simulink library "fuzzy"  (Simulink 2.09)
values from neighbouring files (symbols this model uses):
  a = -1    [HdataM.m]
  alpha = 4    [VdataM.m]
  b = 1    [HdataM.m]
  ce_n = [-1 -0.5 0 0.5 1]    [HdataF.m]    (also in Mdata.m = e_n; Mdata25.m = e_n; VdataF.m = e_n; VdataF25.m = e_n)
  ceNorm = 0.033    [HdataF.m]    (also in Mdata.m = 1; Mdata25.m = 1; VdataF.m = 0.2; VdataF25.m = 0.2)
  e_n = [-1 -0.5 0 0.5 1]    [HdataF.m]    (also in Mdata.m = [-1 -0.25 0 0.25 1]; Mdata25.m = [-1 -0.5 -0.25 0 0.25 0.5 1]; VdataF.m = [-1 -0.25 0 0.25 1]; VdataF25.m = [-1 -0.5 -0.25 0 0.25 0.5 1])
  eNorm = 0.033    [HdataF.m]    (also in Mdata.m = 1; Mdata25.m = 1; VdataF.m = 0.1; VdataF25.m = 0.1)
  Fe0 = Fi+gamma*sqrt(theta0)    [VdataM.m]
  Fg = 0    [VdataM.m]
  Fi = 1000    [VdataM.m]
  gamma = 12500    [VdataM.m]
  gamma1 = 0    [VdataM.m]
  gamma3 = 0    [VdataM.m]
  LN = [1 1 0 0 0 0 0]    [Mdata25.m]    (also in VdataF25.m)
  LP = [0 0 0 0 0 1 1]    [Mdata25.m]    (also in VdataF25.m)
  m = 1000    [VdataM.m]
  N = [1 1 0 0 0]    [HdataF.m]    (also in Mdata.m; VdataF.m)
  P = [0 0 0 1 1]    [HdataF.m]    (also in Mdata.m; VdataF.m)
  Qt = 10    [HdataM.m]
  SN = [0 0 1 0 0 0 0]    [Mdata25.m]    (also in VdataF25.m)
  SP = [0 0 0 0 1 0 0]    [Mdata25.m]    (also in VdataF25.m)
  T = 2.5    [HdataF.m]    (also in Mdata.m = 0.5; Mdata25.m = 0.5; VdataC.m = 0.25; VdataF.m = 0.25)
  T0 = 50    [HdataM.m]
  Tc = 0    [HdataM.m]
  te_n = 0.1    [VdataM.m]
  te_p = 1    [VdataM.m]
  Th = 100    [HdataM.m]
  theta0 = ((1/gamma)*(alpha*v0^2-Fi))^2    (= 0.186624)    [VdataM.m]
  thetamax = pi/3    (= 1.0471975512)    [VdataM.m]
  u0 = 0    [HdataF.m]    (also in Mdata.m; Mdata25.m; VdataF.m = theta0; VdataF25.m = theta0)
  uDenorm = 0.05    [HdataF.m]    (also in Mdata.m = 1; Mdata25.m = 1; VdataF.m = 0.1; VdataF25.m = 0.1)
  uLN = -1    [Mdata25.m]    (also in VdataF25.m)
  uLP = 1    [Mdata25.m]    (also in VdataF25.m)
  uN = -1    [Mdata.m]    (also in VdataF.m)
  uP = 1    [Mdata.m]    (also in VdataF.m)
  uSN = -0.5    [Mdata25.m]    (also in VdataF25.m)
  uSP = 0.5    [Mdata25.m]    (also in VdataF25.m)
  uZ = 0    [Mdata.m]    (also in Mdata25.m; VdataF.m; VdataF25.m)
  v0 = 40    [VdataM.m]
  Z = [0 0 1 0 0]    [HdataF.m]    (also in Mdata.m; Mdata25.m = [0 0 0 1 0 0 0]; VdataF.m; VdataF25.m = [0 0 0 1 0 0 0])
undefined symbols (not defined in the file or in its folder): i1, i2, nb, nm, pb, pm, x, ze, zi
libraries: fuzzy x6
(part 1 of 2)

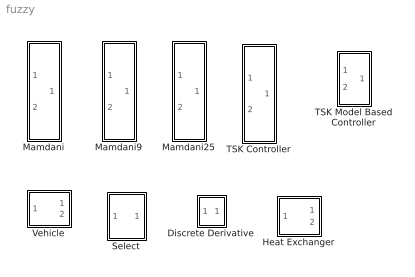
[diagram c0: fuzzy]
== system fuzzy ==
  Discrete Derivative : Subsystem
  Heat Exchanger : Subsystem
  Mamdani : Subsystem
  Mamdani25 : Subsystem
  Mamdani9 : Subsystem
  Select : Subsystem
  TSK Controller : Subsystem
  TSK Model Based Controller : Subsystem
  Vehicle : Subsystem

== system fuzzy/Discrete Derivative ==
  e : Inport  Port=1  PortWidth=-1  SampleTime=-1
  Sum1 : Sum  Inputs=+-
  Unit Delay : UnitDelay  X0=0  SampleTime=T
  ce : Outport  Port=1  InitialOutput=0
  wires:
  e/1 -> Unit Delay/1, Sum1/1
  Sum1/1 -> ce/1
  Unit Delay/1 -> Sum1/2

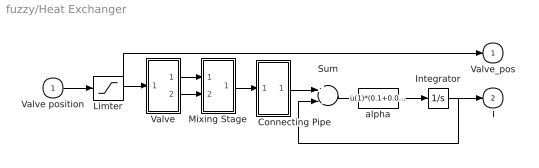
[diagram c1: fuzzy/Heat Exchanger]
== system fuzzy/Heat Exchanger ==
  Valve position : Inport  Port=1  PortWidth=-1  SampleTime=-1
  Connecting Pipe : Subsystem
  Integrator : Integrator  ExternalReset=none  InitialConditionSource=internal  InitialCondition=T0  LimitOutput=off  UpperSaturationLimit=inf  LowerSaturationLimit=-inf  ShowSaturationPort=off  ShowStatePort=off  AbsoluteTolerance=auto
  Limter : Saturate  UpperLimit=1  LowerLimit=-1
  Mixing Stage : Subsystem
  Sum : Sum  Inputs=+-
  Valve : Subsystem
  alpha : Fcn  Expr=u(1)*(0.1+0.01*abs(u(1)))
  Valve_pos : Outport  Port=1  InitialOutput=0
  T : Outport  Port=2  InitialOutput=0
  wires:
  Limter/1 -> Valve_pos/1, Valve/1(Valve_position)
  alpha/1 -> Integrator/1
  Integrator/1 -> T/1, Sum/2
  Valve position/1 -> Limter/1
  Valve/2(Qc) -> Mixing Stage/2(Qc)
  Valve/1(Qh) -> Mixing Stage/1(Qh)
  Mixing Stage/1(Tm) -> Connecting Pipe/1(Tm)
  Sum/1 -> alpha/1
  Connecting Pipe/1(Tf) -> Sum/1

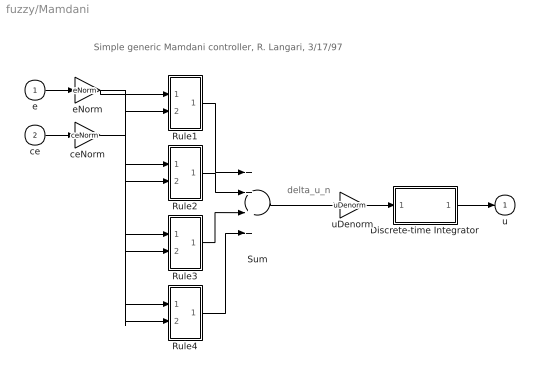
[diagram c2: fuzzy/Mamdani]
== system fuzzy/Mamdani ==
  note: Simple generic Mamdani controller, R. Langari, 3/17/97
  note: delta_u_n
  e : Inport  Port=1  PortWidth=-1  SampleTime=-1
  ce : Inport  Port=2  PortWidth=-1  SampleTime=-1
  Discrete-time Integrator : Subsystem
  Rule1 : Subsystem
  Rule2 : Subsystem
  Rule3 : Subsystem
  Rule4 : Subsystem
  Sum : Sum  Inputs=++++
  ceNorm : Gain  Gain=ceNorm
  eNorm : Gain  Gain=eNorm
  uDenorm : Gain  Gain=uDenorm
  u : Outport  Port=1  InitialOutput=0
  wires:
  ce/1 -> ceNorm/1
  e/1 -> eNorm/1
  eNorm/1 -> Rule2/1(e_n), Rule3/1(e_n), Rule4/1(e_n), Rule1/1(e_n)
  ceNorm/1 -> Rule1/2(ce_n), Rule2/2(ce_n), Rule3/2(ce_n), Rule4/2(ce_n)
  Rule1/1(delta_u_n) -> Sum/1
  Rule2/1(delta_u_n) -> Sum/2
  Rule3/1(delta_u_n) -> Sum/3
  Rule4/1(delta_u_n) -> Sum/4
  Sum/1 -> uDenorm/1
  uDenorm/1 -> Discrete-time Integrator/1(delta_u)
  Discrete-time Integrator/1(u) -> u/1

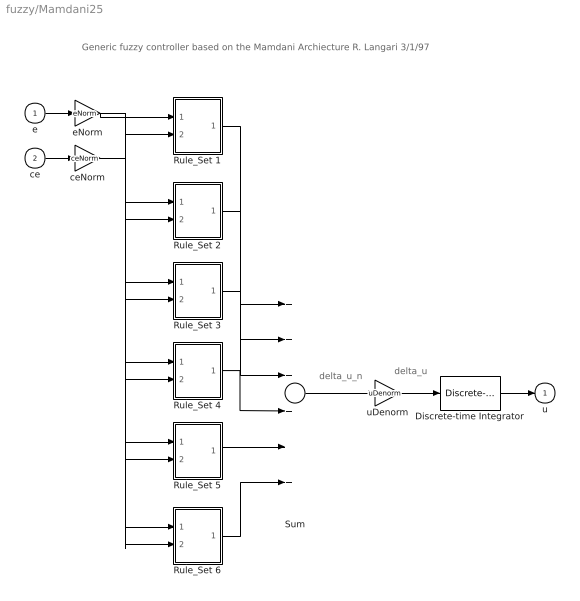
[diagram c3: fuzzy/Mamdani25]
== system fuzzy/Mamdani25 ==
  note: Generic fuzzy controller based on the Mamdani Archiecture R. Langari 3/1/97
  note: delta_u_n
  note: delta_u
  e : Inport  Port=1  PortWidth=-1  SampleTime=-1
  ce : Inport  Port=2  PortWidth=-1  SampleTime=-1
  Discrete-time Integrator : fuzzy/Mamdani/Discrete-time Integrator
  Rule_Set 1 : Subsystem
  Rule_Set 2 : Subsystem
  Rule_Set 3 : Subsystem
  Rule_Set 4 : Subsystem
  Rule_Set 5 : Subsystem
  Rule_Set 6 : Subsystem
  Sum : Sum  Inputs=++++++
  ceNorm : Gain  Gain=ceNorm
  eNorm : Gain  Gain=eNorm
  uDenorm : Gain  Gain=uDenorm
  u : Outport  Port=1  InitialOutput=0
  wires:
  Rule_Set 6/1(delta_u_n) -> Sum/6
  Rule_Set 5/1(delta_u_n) -> Sum/5
  Rule_Set 4/1(delta_u_n) -> Sum/4
  Rule_Set 3/1(delta_u_n) -> Sum/3
  Rule_Set 2/1(delta_u_n) -> Sum/2
  Rule_Set 1/1(delta_u_n) -> Sum/1
  ceNorm/1 -> Rule_Set 5/2(ce_n), Rule_Set 6/2(ce_n), Rule_Set 4/2(ce_n), Rule_Set 3/2(ce_n), Rule_Set 2/2(ce_n), Rule_Set 1/2(ce_n)
  eNorm/1 -> Rule_Set 6/1(e_n), Rule_Set 5/1(e_n), Rule_Set 4/1(e_n), Rule_Set 3/1(e_n), Rule_Set 2/1(e_n), Rule_Set 1/1(e_n)
  uDenorm/1 -> Discrete-time Integrator/1
  Sum/1 -> uDenorm/1
  ce/1 -> ceNorm/1
  e/1 -> eNorm/1
  Discrete-time Integrator/1 -> u/1

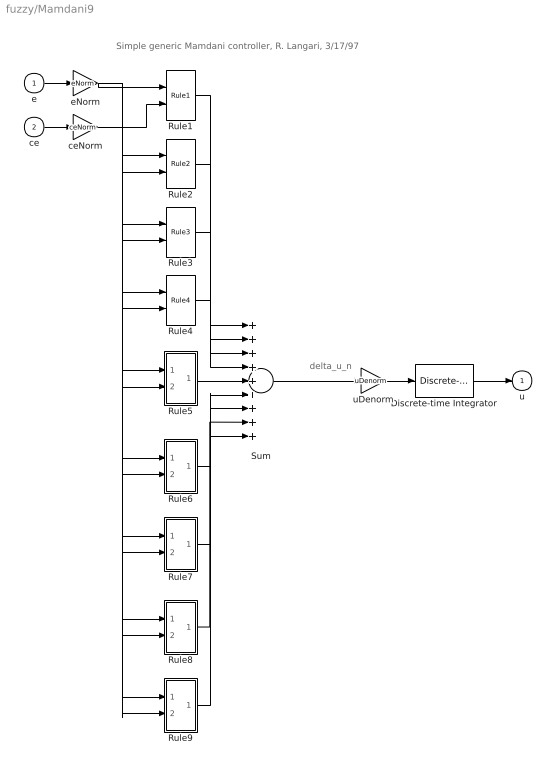
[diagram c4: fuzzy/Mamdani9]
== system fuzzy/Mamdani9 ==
  note: Simple generic Mamdani controller, R. Langari, 3/17/97
  note: delta_u_n
  e : Inport  Port=1  PortWidth=-1  SampleTime=-1
  ce : Inport  Port=2  PortWidth=-1  SampleTime=-1
  Discrete-time Integrator : fuzzy/Mamdani/Discrete-time Integrator
  Rule1 : fuzzy/Mamdani/Rule1
  Rule2 : fuzzy/Mamdani/Rule2
  Rule3 : fuzzy/Mamdani/Rule3
  Rule4 : fuzzy/Mamdani/Rule4
  Rule5 : Subsystem
  Rule6 : Subsystem
  Rule7 : Subsystem
  Rule8 : Subsystem
  Rule9 : Subsystem
  Sum : Sum  Inputs=+++++++++
  ceNorm : Gain  Gain=ceNorm
  eNorm : Gain  Gain=eNorm
  uDenorm : Gain  Gain=uDenorm
  u : Outport  Port=1  InitialOutput=0
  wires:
  Rule4/1 -> Sum/4
  Rule3/1 -> Sum/3
  Rule2/1 -> Sum/2
  Rule1/1 -> Sum/1
  ceNorm/1 -> Rule3/2, Rule2/2, Rule1/2, Rule4/2, Rule5/2(ce_n), Rule6/2(ce_n), Rule7/2(ce_n), Rule8/2(ce_n), Rule9/2(ce_n)
  eNorm/1 -> Rule3/1, Rule2/1, Rule4/1, Rule5/1(e_n), Rule6/1(e_n), Rule7/1(e_n), Rule8/1(e_n), Rule9/1(e_n), Rule1/1
  e/1 -> eNorm/1
  ce/1 -> ceNorm/1
  Rule5/1(delta_u_n) -> Sum/5
  Rule6/1(delta_u_n) -> Sum/6
  Rule7/1(delta_u_n) -> Sum/7
  Rule8/1(delta_u_n) -> Sum/8
  Rule9/1(delta_u_n) -> Sum/9
  uDenorm/1 -> Discrete-time Integrator/1
  Discrete-time Integrator/1 -> u/1
  Sum/1 -> uDenorm/1

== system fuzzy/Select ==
  theta_in : Inport  Port=1  PortWidth=-1  SampleTime=-1
  Manual mode throttle position : Constant  Value=theta0
  On/Off : Constant  Value=1
  Switch : Switch  Threshold=0.5
  theta_out : Outport  Port=1  InitialOutput=0
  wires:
  Switch/1 -> theta_out/1
  theta_in/1 -> Switch/1
  Manual mode throttle position/1 -> Switch/3
  On/Off/1 -> Switch/2

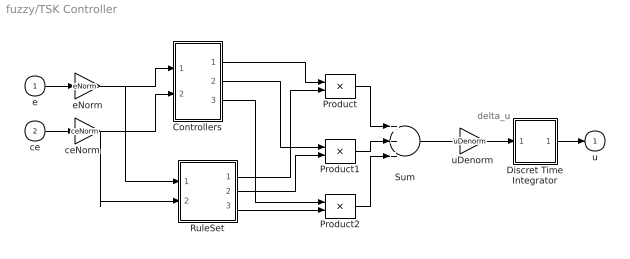
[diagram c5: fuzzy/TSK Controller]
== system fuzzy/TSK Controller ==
  note: delta_u
  e : Inport  Port=1  PortWidth=-1  SampleTime=-1
  ce : Inport  Port=2  PortWidth=-1  SampleTime=-1
  Controllers : Subsystem
  Discret Time Integrator : Subsystem  mask(Discrete-Time Integrator){}
      mask help: Discrete-Time Integrator:
      mask init:
      | X0=@1;Ts=@2;
  Product : Product  Inputs=2
  Product1 : Product  Inputs=2
  Product2 : Product  Inputs=2
  RuleSet : Subsystem
  Sum : Sum  Inputs=+++
  ceNorm : Gain  Gain=ceNorm
  eNorm : Gain  Gain=eNorm
  uDenorm : Gain  Gain=uDenorm
  u : Outport  Port=1  InitialOutput=0
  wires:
  Sum/1 -> uDenorm/1
  Discret Time Integrator/1(out_1) -> u/1
  uDenorm/1 -> Discret Time Integrator/1(in_1)
  ceNorm/1 -> Controllers/2(ce_n), RuleSet/2(ce)
  eNorm/1 -> Controllers/1(e_n), RuleSet/1(e)
  e/1 -> eNorm/1
  ce/1 -> ceNorm/1
  Product1/1 -> Sum/2
  Product/1 -> Sum/1
  RuleSet/2(w2) -> Product1/2
  Controllers/2(delta_u_n2) -> Product1/1
  RuleSet/1(w1) -> Product/2
  Controllers/1(delta_u_n1) -> Product/1
  Controllers/3(delta_u_n3) -> Product2/1
  RuleSet/3(w3) -> Product2/2
  Product2/1 -> Sum/3

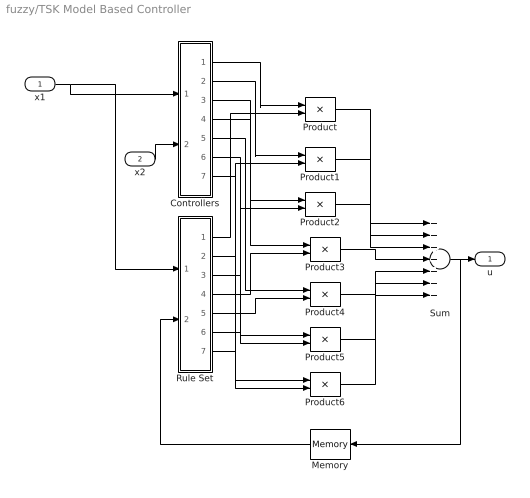
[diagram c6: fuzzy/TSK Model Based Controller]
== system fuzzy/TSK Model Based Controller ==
  x1 : Inport  Port=1  PortWidth=-1  SampleTime=-1
  x2 : Inport  Port=2  PortWidth=-1  SampleTime=-1
  Controllers : Subsystem
  Memory : Memory  Orientation=left  X0=0  InheritSampleTime=off
  Product{,1..6} (7 alike) : Product  Inputs=2
  Rule Set : Subsystem
  Sum : Sum  Inputs=+++++++
  u : Outport  Port=1  InitialOutput=0
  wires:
  Sum/1 -> Memory/1, u/1
  Controllers/1(out_1) -> Product/1
  Rule Set/1(out_1) -> Product/2
  Controllers/2(out_2) -> Product1/1
  Controllers/3(out_3) -> Product2/1
  Controllers/4(out_4) -> Product3/1
  Controllers/5(out_5) -> Product4/1
  Controllers/6(out_6) -> Product5/1
  Controllers/7(out_7) -> Product6/1
  Rule Set/2(out_2) -> Product1/2
  Rule Set/3(out_3) -> Product2/2
  Rule Set/4(out_4) -> Product3/2
  Rule Set/5(out_5) -> Product4/2
  Rule Set/6(out_6) -> Product5/2
  Rule Set/7(out_7) -> Product6/2
  Product/1 -> Sum/1
  Product1/1 -> Sum/2
  Product2/1 -> Sum/3
  Product3/1 -> Sum/4
  Product4/1 -> Sum/5
  Product5/1 -> Sum/6
  Product6/1 -> Sum/7
  x1/1 -> Controllers/1(x1), Rule Set/1(x1)
  Memory/1 -> Rule Set/2(x2)
  x2/1 -> Controllers/2(x2)

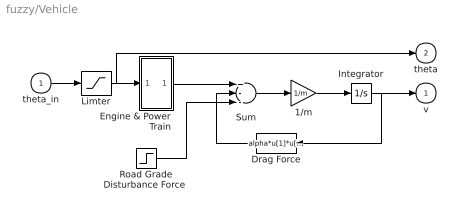
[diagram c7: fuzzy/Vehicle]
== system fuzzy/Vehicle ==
  theta_in : Inport  Port=1  PortWidth=-1  SampleTime=-1
  1/m : Gain  Gain=1/m
  Drag Force : Fcn  Orientation=left  Expr=alpha*u[1]*u[1]
  Engine & Power Train : Subsystem
  Integrator : Integrator  ExternalReset=none  InitialConditionSource=internal  InitialCondition=v0  LimitOutput=off  UpperSaturationLimit=inf  LowerSaturationLimit=-inf  ShowSaturationPort=off  ShowStatePort=off  AbsoluteTolerance=auto
  Limter : Saturate  UpperLimit=thetamax  LowerLimit=0
  "Road Grade Disturbance Force " : Step  Time=0  Before=0  After=Fg
  Sum : Sum  Inputs=+--
  v : Outport  Port=1  InitialOutput=0
  theta : Outport  Port=2  InitialOutput=0
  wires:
  Limter/1 -> theta/1, Engine & Power Train/1(theta)
  "Road Grade Disturbance Force "/1 -> Sum/3
  theta_in/1 -> Limter/1
  Sum/1 -> 1/m/1
  1/m/1 -> Integrator/1
  Integrator/1 -> Drag Force/1, v/1
  Engine & Power Train/1(Engine Force_) -> Sum/1
  Drag Force/1 -> Sum/2

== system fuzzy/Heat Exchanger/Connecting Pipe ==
  Tm : Inport  Port=1  PortWidth=-1  SampleTime=-1
  Integrator : Integrator  ExternalReset=none  InitialConditionSource=internal  InitialCondition=T0  LimitOutput=off  UpperSaturationLimit=inf  LowerSaturationLimit=-inf  ShowSaturationPort=off  ShowStatePort=off  AbsoluteTolerance=auto
  Sum : Sum  Inputs=++
  a : Gain  Orientation=left  Gain=a
  b : Gain  Gain=b
  Tf : Outport  Port=1  InitialOutput=0
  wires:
  a/1 -> Sum/2
  Integrator/1 -> a/1, Tf/1
  b/1 -> Sum/1
  Sum/1 -> Integrator/1
  Tm/1 -> b/1

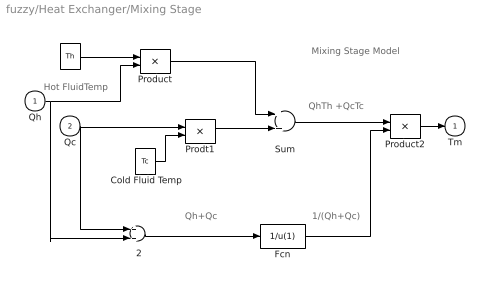
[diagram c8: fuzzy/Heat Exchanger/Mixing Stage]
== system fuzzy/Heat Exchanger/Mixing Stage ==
  note: Mixing Stage Model
  note: 1/(Qh+Qc)
  note: Qh+Qc
  note: QhTh +QcTc
  note: Hot FluidTemp
  Qh : Inport  Port=1  PortWidth=-1  SampleTime=-1
  Qc : Inport  Port=2  PortWidth=-1  SampleTime=-1
  " " : Constant  Value=Th
  " 2" : Sum  Inputs=++
  " Cold Fluid Temp" : Constant  Value=Tc
  Fcn : Fcn  Expr=1/u(1)
  Prodt1 : Product  Inputs=2
  Product : Product  Inputs=2
  Product2 : Product  Inputs=2
  Sum : Sum  Inputs=++
  Tm : Outport  Port=1  InitialOutput=0
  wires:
  Fcn/1 -> Product2/2
  Sum/1 -> Product2/1
  Qh/1 -> " 2"/2, Product/2
  Qc/1 -> " 2"/1, Prodt1/1
  " Cold Fluid Temp"/1 -> Prodt1/2
  " 2"/1 -> Fcn/1
  Prodt1/1 -> Sum/2
  Product/1 -> Sum/1
  " "/1 -> Product/1
  Product2/1 -> Tm/1

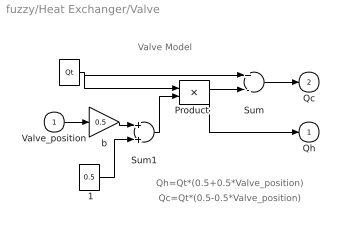
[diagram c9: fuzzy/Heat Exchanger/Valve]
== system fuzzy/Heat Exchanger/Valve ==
  note: Qc=Qt*(0.5-0.5*Valve_position)
  note: Qh=Qt*(0.5+0.5*Valve_position)
  note: Valve Model
  Valve_position : Inport  Port=1  PortWidth=-1  SampleTime=-1
  " " : Constant  Value=Qt
  " 1" : Constant  Value=0.5
  Product : Product  Inputs=2
  Sum : Sum  Inputs=+-
  Sum1 : Sum  Inputs=++
  b : Gain  Gain=0.5
  Qh : Outport  Port=1  InitialOutput=0
  Qc : Outport  Port=2  InitialOutput=0
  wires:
  Sum1/1 -> Product/2
  " 1"/1 -> Sum1/2
  b/1 -> Sum1/1
  Valve_position/1 -> b/1
  Product/1 -> Sum/2, Qh/1
  Sum/1 -> Qc/1
  " "/1 -> Sum/1, Product/1

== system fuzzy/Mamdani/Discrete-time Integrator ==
  delta_u : Inport  Port=1  PortWidth=-1  SampleTime=-1
  Sum : Sum  Inputs=++
  Unit Delay : UnitDelay  Orientation=left  X0=u0  SampleTime=T
  u : Outport  Port=1  InitialOutput=0
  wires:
  Unit Delay/1 -> Sum/2
  Sum/1 -> u/1, Unit Delay/1
  delta_u/1 -> Sum/1

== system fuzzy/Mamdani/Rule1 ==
  note: if e_n is P and ce_n is P then delta_u_n is P
  e_n : Inport  Port=1  PortWidth=-1  SampleTime=-1
  ce_n : Inport  Port=2  PortWidth=-1  SampleTime=-1
  P(ce_n) : Lookup  InputValues=ce_n  OutputValues=P
  P(delta_u_n) : Constant  Value=uP
  P(e_n) : Lookup  InputValues=e_n  OutputValues=P
  Product : Product  Inputs=2
  Product1 : Product  Inputs=2
  delta_u_n : Outport  Port=1  InitialOutput=0
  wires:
  Product/1 -> Product1/1
  ce_n/1 -> P(ce_n)/1
  P(ce_n)/1 -> Product/2
  P(delta_u_n)/1 -> Product1/2
  e_n/1 -> P(e_n)/1
  P(e_n)/1 -> Product/1
  Product1/1 -> delta_u_n/1

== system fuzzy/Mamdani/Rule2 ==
  note: if e_n is P and ce_n is N then delta_u_n is Z
  e_n : Inport  Port=1  PortWidth=-1  SampleTime=-1
  ce_n : Inport  Port=2  PortWidth=-1  SampleTime=-1
  N(ce_n) : Lookup  InputValues=ce_n  OutputValues=N
  P(e_n) : Lookup  InputValues=e_n  OutputValues=P
  Prduct : Product  Inputs=2
  Product1 : Product  Inputs=2
  Z(delta_u_n) : Constant  Value=uZ
  delta_u_n : Outport  Port=1  InitialOutput=0
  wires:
  Product1/1 -> delta_u_n/1
  Z(delta_u_n)/1 -> Product1/2
  Prduct/1 -> Product1/1
  P(e_n)/1 -> Prduct/1
  N(ce_n)/1 -> Prduct/2
  e_n/1 -> P(e_n)/1
  ce_n/1 -> N(ce_n)/1

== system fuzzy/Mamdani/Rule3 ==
  note: if e_n is N and ce_n is P then delta_u_n is Z
  e_n : Inport  Port=1  PortWidth=-1  SampleTime=-1
  ce_n : Inport  Port=2  PortWidth=-1  SampleTime=-1
  N(e_n) : Lookup  InputValues=e_n  OutputValues=N
  P(ce_n) : Lookup  InputValues=ce_n  OutputValues=P
  Product : Product  Inputs=2
  Product1 : Product  Inputs=2
  Z(delta_u_n) : Constant  Value=uZ
  delta_u_n : Outport  Port=1  InitialOutput=0
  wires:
  ce_n/1 -> P(ce_n)/1
  e_n/1 -> N(e_n)/1
  P(ce_n)/1 -> Product/2
  N(e_n)/1 -> Product/1
  Product/1 -> Product1/1
  Z(delta_u_n)/1 -> Product1/2
  Product1/1 -> delta_u_n/1

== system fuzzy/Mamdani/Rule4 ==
  note: if e_n is N and ce_n is N then delta_u_n is N
  e_n : Inport  Port=1  PortWidth=-1  SampleTime=-1
  ce_n : Inport  Port=2  PortWidth=-1  SampleTime=-1
  N(ce_n) : Lookup  InputValues=ce_n  OutputValues=N
  N(delta_u_n) : Constant  Value=uN
  N(e_n) : Lookup  InputValues=e_n  OutputValues=N
  Product : Product  Inputs=2
  Product1 : Product  Inputs=2
  delta_u_n : Outport  Port=1  InitialOutput=0
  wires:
  Product1/1 -> delta_u_n/1
  N(delta_u_n)/1 -> Product1/2
  Product/1 -> Product1/1
  N(e_n)/1 -> Product/1
  N(ce_n)/1 -> Product/2
  e_n/1 -> N(e_n)/1
  ce_n/1 -> N(ce_n)/1

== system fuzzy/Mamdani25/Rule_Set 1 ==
  e_n : Inport  Port=1  PortWidth=-1  SampleTime=-1
  ce_n : Inport  Port=2  PortWidth=-1  SampleTime=-1
  Rule1 : Subsystem
  Rule2 : Subsystem
  Rule3 : Subsystem
  Rule4 : Subsystem
  Sum : Sum  Inputs=++++
  delta_u_n : Outport  Port=1  InitialOutput=0
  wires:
  Sum/1 -> delta_u_n/1
  Rule4/1(delta_u_n) -> Sum/4
  Rule3/1(delta_u_n) -> Sum/3
  Rule2/1(delta_u_n) -> Sum/2
  Rule1/1(delta_u_n) -> Sum/1
  e_n/1 -> Rule4/1(e_n), Rule3/1(e_n), Rule2/1(e_n), Rule1/1(e_n)
  ce_n/1 -> Rule4/2(ce_n), Rule3/2(ce_n), Rule2/2(ce_n), Rule1/2(ce_n)

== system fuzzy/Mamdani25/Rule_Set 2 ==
  e_n : Inport  Port=1  PortWidth=-1  SampleTime=-1
  ce_n : Inport  Port=2  PortWidth=-1  SampleTime=-1
  Rule1 : Subsystem
  Rule2 : Subsystem
  Rule3 : Subsystem
  Rule4 : Subsystem
  Sum : Sum  Inputs=++++
  delta_u_n : Outport  Port=1  InitialOutput=0
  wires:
  Rule1/1(delta_u_n) -> Sum/1
  Rule2/1(delta_u_n) -> Sum/2
  Rule3/1(delta_u_n) -> Sum/3
  Rule4/1(delta_u_n) -> Sum/4
  Sum/1 -> delta_u_n/1
  e_n/1 -> Rule1/1(e_n), Rule2/1(e_n), Rule3/1(e_n), Rule4/1(e_n)
  ce_n/1 -> Rule1/2(ce_n), Rule2/2(ce_n), Rule3/2(ce_n), Rule4/2(ce_n)

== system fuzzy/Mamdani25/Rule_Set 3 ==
  e_n : Inport  Port=1  PortWidth=-1  SampleTime=-1
  ce_n : Inport  Port=2  PortWidth=-1  SampleTime=-1
  Rule1 : Subsystem
  Rule2 : Subsystem
  Rule3 : Subsystem
  Rule4 : Subsystem
  Sum : Sum  Inputs=++++
  delta_u_n : Outport  Port=1  InitialOutput=0
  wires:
  Sum/1 -> delta_u_n/1
  Rule4/1(delta_u_n) -> Sum/4
  Rule3/1(delta_u_n) -> Sum/3
  Rule2/1(delta_u_n) -> Sum/2
  Rule1/1(delta_u_n) -> Sum/1
  e_n/1 -> Rule4/1(e_n), Rule3/1(e_n), Rule2/1(e_n), Rule1/1(e_n)
  ce_n/1 -> Rule4/2(ce_n), Rule3/2(ce_n), Rule2/2(ce_n), Rule1/2(ce_n)

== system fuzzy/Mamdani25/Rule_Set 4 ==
  e_n : Inport  Port=1  PortWidth=-1  SampleTime=-1
  ce_n : Inport  Port=2  PortWidth=-1  SampleTime=-1
  Rule1 : Subsystem
  Rule2 : Subsystem
  Rule3 : Subsystem
  Rule4 : Subsystem
  Sum : Sum  Inputs=++++
  delta_u_n : Outport  Port=1  InitialOutput=0
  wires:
  Rule1/1(delta_u_n) -> Sum/1
  Rule2/1(delta_u_n) -> Sum/2
  Rule3/1(delta_u_n) -> Sum/3
  Rule4/1(delta_u_n) -> Sum/4
  Sum/1 -> delta_u_n/1
  e_n/1 -> Rule1/1(e_n), Rule2/1(e_n), Rule3/1(e_n), Rule4/1(e_n)
  ce_n/1 -> Rule1/2(ce_n), Rule2/2(ce_n), Rule3/2(ce_n), Rule4/2(ce_n)

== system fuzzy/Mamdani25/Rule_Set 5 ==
  e_n : Inport  Port=1  PortWidth=-1  SampleTime=-1
  ce_n : Inport  Port=2  PortWidth=-1  SampleTime=-1
  Rule1 : Subsystem
  Rule2 : Subsystem
  Rule3 : Subsystem
  Rule4 : Subsystem
  Sum : Sum  Inputs=++++
  delta_u_n : Outport  Port=1  InitialOutput=0
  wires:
  Sum/1 -> delta_u_n/1
  Rule4/1(delta_u_n) -> Sum/4
  Rule3/1(delta_u_n) -> Sum/3
  Rule2/1(delta_u_n) -> Sum/2
  Rule1/1(delta_u_n) -> Sum/1
  e_n/1 -> Rule4/1(e_n), Rule3/1(e_n), Rule2/1(e_n), Rule1/1(e_n)
  ce_n/1 -> Rule4/2(ce_n), Rule3/2(ce_n), Rule2/2(ce_n), Rule1/2(ce_n)

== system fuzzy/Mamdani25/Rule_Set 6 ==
  e_n : Inport  Port=1  PortWidth=-1  SampleTime=-1
  ce_n : Inport  Port=2  PortWidth=-1  SampleTime=-1
  Rule1 : Subsystem
  Rule2 : Subsystem
  Rule3 : Subsystem
  Rule4 : Subsystem
  Rule5 : Subsystem
  Sum : Sum  Inputs=+++++
  delta_u_n : Outport  Port=1  InitialOutput=0
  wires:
  Rule5/1(delta_u_n) -> Sum/5
  Rule1/1(delta_u_n) -> Sum/1
  Rule2/1(delta_u_n) -> Sum/2
  Rule3/1(delta_u_n) -> Sum/3
  Rule4/1(delta_u_n) -> Sum/4
  Sum/1 -> delta_u_n/1
  e_n/1 -> Rule5/1(e_n), Rule1/1(e_n), Rule2/1(e_n), Rule3/1(e_n), Rule4/1(e_n)
  ce_n/1 -> Rule5/2(ce_n), Rule1/2(ce_n), Rule2/2(ce_n), Rule3/2(ce_n), Rule4/2(ce_n)

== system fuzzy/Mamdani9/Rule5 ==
  note: if e_n is P and ce_n is Z then delta_u_n is P
  e_n : Inport  Port=1  PortWidth=-1  SampleTime=-1
  ce_n : Inport  Port=2  PortWidth=-1  SampleTime=-1
  P(delta_u_n) : Constant  Value=uP
  P(e_n) : Lookup  InputValues=e_n  OutputValues=P
  Product : Product  Inputs=2
  Product1 : Product  Inputs=2
  Z(ce_n) : Lookup  InputValues=ce_n  OutputValues=Z
  delta_u_n : Outport  Port=1  InitialOutput=0
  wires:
  Product/1 -> Product1/1
  ce_n/1 -> Z(ce_n)/1
  Z(ce_n)/1 -> Product/2
  P(delta_u_n)/1 -> Product1/2
  e_n/1 -> P(e_n)/1
  P(e_n)/1 -> Product/1
  Product1/1 -> delta_u_n/1

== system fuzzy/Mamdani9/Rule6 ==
  note: if e_n is N and ce_n is Z then delta_u_n is N
  e_n : Inport  Port=1  PortWidth=-1  SampleTime=-1
  ce_n : Inport  Port=2  PortWidth=-1  SampleTime=-1
  N(delta_u_n) : Constant  Value=uN
  N(e_n) : Lookup  InputValues=e_n  OutputValues=N
  Product : Product  Inputs=2
  Product1 : Product  Inputs=2
  Z(ce_n) : Lookup  InputValues=ce_n  OutputValues=Z
  delta_u_n : Outport  Port=1  InitialOutput=0
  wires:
  Product1/1 -> delta_u_n/1
  N(delta_u_n)/1 -> Product1/2
  Product/1 -> Product1/1
  N(e_n)/1 -> Product/1
  Z(ce_n)/1 -> Product/2
  e_n/1 -> N(e_n)/1
  ce_n/1 -> Z(ce_n)/1

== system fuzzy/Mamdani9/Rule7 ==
  note: if e_n is Z and ce_n is P then delta_u_n is P
  e_n : Inport  Port=1  PortWidth=-1  SampleTime=-1
  ce_n : Inport  Port=2  PortWidth=-1  SampleTime=-1
  P(ce_n) : Lookup  InputValues=ce_n  OutputValues=P
  P(delta_u_n) : Constant  Value=uP
  Product : Product  Inputs=2
  Product1 : Product  Inputs=2
  Z(e_n) : Lookup  InputValues=e_n  OutputValues=Z
  delta_u_n : Outport  Port=1  InitialOutput=0
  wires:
  ce_n/1 -> P(ce_n)/1
  e_n/1 -> Z(e_n)/1
  P(ce_n)/1 -> Product/2
  Z(e_n)/1 -> Product/1
  Product/1 -> Product1/1
  P(delta_u_n)/1 -> Product1/2
  Product1/1 -> delta_u_n/1

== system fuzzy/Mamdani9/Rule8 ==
  note: if e_n is Z and ce_n is N then delta_u_n is N
  e_n : Inport  Port=1  PortWidth=-1  SampleTime=-1
  ce_n : Inport  Port=2  PortWidth=-1  SampleTime=-1
  N(ce_n) : Lookup  InputValues=ce_n  OutputValues=N
  N(delta_u_n) : Constant  Value=uN
  Prduct : Product  Inputs=2
  Z(e_n) : Lookup  InputValues=e_n  OutputValues=Z
  roduct1 : Product  Inputs=2
  delta_u_n : Outport  Port=1  InitialOutput=0
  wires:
  roduct1/1 -> delta_u_n/1
  N(delta_u_n)/1 -> roduct1/2
  Prduct/1 -> roduct1/1
  Z(e_n)/1 -> Prduct/1
  N(ce_n)/1 -> Prduct/2
  e_n/1 -> Z(e_n)/1
  ce_n/1 -> N(ce_n)/1

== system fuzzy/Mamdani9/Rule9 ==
  note: if e_n is Z and ce_n is Z then delta_u_n is Z
  e_n : Inport  Port=1  PortWidth=-1  SampleTime=-1
  ce_n : Inport  Port=2  PortWidth=-1  SampleTime=-1
  P(e_n) : Lookup  InputValues=e_n  OutputValues=Z
  Product : Product  Inputs=2
  Product1 : Product  Inputs=2
  Z(ce_n) : Lookup  InputValues=ce_n  OutputValues=Z
  Z(delta_u_n) : Constant  Value=uZ
  delta_u_n : Outport  Port=1  InitialOutput=0
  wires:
  Product1/1 -> delta_u_n/1
  P(e_n)/1 -> Product/1
  e_n/1 -> P(e_n)/1
  Z(delta_u_n)/1 -> Product1/2
  Z(ce_n)/1 -> Product/2
  ce_n/1 -> Z(ce_n)/1
  Product/1 -> Product1/1

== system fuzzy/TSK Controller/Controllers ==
  e_n : Inport  Port=1  PortWidth=-1  SampleTime=-1
  ce_n : Inport  Port=2  PortWidth=-1  SampleTime=-1
  SF1 : Subsystem  mask(StateFeedback){}
      mask help: Gains
      mask init:
      | K1=@1;K2=@2;K0=@3;
  SF2 : Subsystem  mask(StateFeedback){}
      mask help: Gains
      mask init:
      | K1=@1;K2=@2;K0=@3;
  SF3 : Subsystem  mask(StateFeedback){}
      mask help: Gains
      mask init:
      | K1=@1;K2=@2;K0=@3;
  delta_u_n1 : Outport  Port=1  InitialOutput=0
  delta_u_n2 : Outport  Port=2  InitialOutput=0
  delta_u_n3 : Outport  Port=3  InitialOutput=0
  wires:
  SF2/1(out_1) -> delta_u_n2/1
  SF1/1(delta_u_n1) -> delta_u_n1/1
  ce_n/1 -> SF1/2(ce_n), SF2/2(in_2), SF3/2(in_2)
  e_n/1 -> SF1/1(e_n), SF2/1(in_1), SF3/1(in_1)
  SF3/1(out_1) -> delta_u_n3/1

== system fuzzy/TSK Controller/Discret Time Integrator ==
  in_1 : Inport  Port=1  PortWidth=-1  SampleTime=-1
  Gain : Gain  Gain=Ts
  Sum : Sum  Inputs=++
  Unit Delay : UnitDelay  X0=X0  SampleTime=Ts
  out_1 : Outport  Port=1  InitialOutput=0
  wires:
  Unit Delay/1 -> Sum/2, out_1/1
  Sum/1 -> Unit Delay/1
  in_1/1 -> Gain/1
  Gain/1 -> Sum/1

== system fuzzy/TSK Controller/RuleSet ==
  e : Inport  Port=1  PortWidth=-1  SampleTime=-1
  ce : Inport  Port=2  PortWidth=-1  SampleTime=-1
  Rule1 : Subsystem
  Rule2 : Subsystem
  Rule3 : Subsystem
  w1 : Outport  Port=1  InitialOutput=0
  w2 : Outport  Port=2  InitialOutput=0
  w3 : Outport  Port=3  InitialOutput=0
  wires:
  Rule2/1(out_1) -> w2/1
  Rule1/1(out_1) -> w1/1
  e/1 -> Rule2/1(in_1), Rule1/1(in_1), Rule3/1(in_1)
  ce/1 -> Rule2/2(in_2), Rule1/2(in_2), Rule3/2(in_2)
  Rule3/1(out_1) -> w3/1

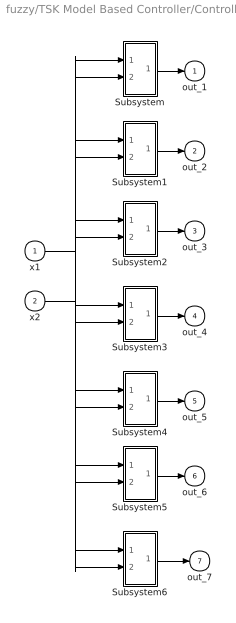
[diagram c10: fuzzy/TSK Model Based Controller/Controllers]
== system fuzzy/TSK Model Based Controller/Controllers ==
  x1 : Inport  Port=1  PortWidth=-1  SampleTime=-1
  x2 : Inport  Port=2  PortWidth=-1  SampleTime=-1
  Subsystem : Subsystem  mask(StateFeedback){}
      mask help: Gains
      mask init:
      | K1=@1;K2=@2;K0=@3;
  Subsystem1 : Subsystem  mask(StateFeedback){}
      mask help: Gains
      mask init:
      | K1=@1;K2=@2;K0=@3;
  Subsystem2 : Subsystem  mask(StateFeedback){}
      mask help: Gains
      mask init:
      | K1=@1;K2=@2;K0=@3;
  Subsystem3 : Subsystem  mask(StateFeedback){}
      mask help: Gains
      mask init:
      | K1=@1;K2=@2;K0=@3;
  Subsystem4 : Subsystem  mask(StateFeedback){}
      mask help: Gains
      mask init:
      | K1=@1;K2=@2;K0=@3;
  Subsystem5 : Subsystem  mask(StateFeedback){}
      mask help: Gains
      mask init:
      | K1=@1;K2=@2;K0=@3;
  Subsystem6 : Subsystem  mask(StateFeedback){}
      mask help: Gains
      mask init:
      | K1=@1;K2=@2;K0=@3;
  out_1 : Outport  Port=1  InitialOutput=0
  out_2 : Outport  Port=2  InitialOutput=0
  out_3 : Outport  Port=3  InitialOutput=0
  out_4 : Outport  Port=4  InitialOutput=0
  out_5 : Outport  Port=5  InitialOutput=0
  out_6 : Outport  Port=6  InitialOutput=0
  out_7 : Outport  Port=7  InitialOutput=0
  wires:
  Subsystem/1(out_1) -> out_1/1
  Subsystem1/1(out_1) -> out_2/1
  Subsystem2/1(out_1) -> out_3/1
  Subsystem3/1(out_1) -> out_4/1
  Subsystem4/1(out_1) -> out_5/1
  Subsystem5/1(out_1) -> out_6/1
  Subsystem6/1(out_1) -> out_7/1
  x1/1 -> Subsystem/1(in_1), Subsystem1/1(in_1), Subsystem2/1(in_1), Subsystem3/1(in_1), Subsystem4/1(in_1), Subsystem5/1(in_1), Subsystem6/1(in_1)
  x2/1 -> Subsystem/2(in_2), Subsystem1/2(in_2), Subsystem4/2(in_2), Subsystem5/2(in_2), Subsystem6/2(in_2), Subsystem3/2(in_2), Subsystem2/2(in_2)

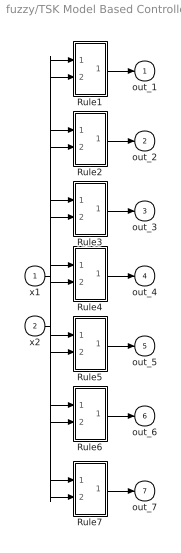
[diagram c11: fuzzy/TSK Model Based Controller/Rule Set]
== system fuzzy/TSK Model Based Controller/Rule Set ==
  x1 : Inport  Port=1  PortWidth=-1  SampleTime=-1
  x2 : Inport  Port=2  PortWidth=-1  SampleTime=-1
  Rule1 : Subsystem
  Rule2 : Subsystem
  Rule3 : Subsystem
  Rule4 : Subsystem
  Rule5 : Subsystem
  Rule6 : Subsystem
  Rule7 : Subsystem
  out_1 : Outport  Port=1  InitialOutput=0
  out_2 : Outport  Port=2  InitialOutput=0
  out_3 : Outport  Port=3  InitialOutput=0
  out_4 : Outport  Port=4  InitialOutput=0
  out_5 : Outport  Port=5  InitialOutput=0
  out_6 : Outport  Port=6  InitialOutput=0
  out_7 : Outport  Port=7  InitialOutput=0
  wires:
  Rule7/1(out_1) -> out_7/1
  Rule6/1(out_1) -> out_6/1
  Rule5/1(out_1) -> out_5/1
  Rule4/1(out_1) -> out_4/1
  Rule3/1(out_1) -> out_3/1
  Rule2/1(out_1) -> out_2/1
  Rule1/1(out_1) -> out_1/1
  x1/1 -> Rule1/1(in_1), Rule2/1(in_1), Rule3/1(in_1), Rule4/1(in_1), Rule5/1(in_1), Rule6/1(in_1), Rule7/1(in_1)
  x2/1 -> Rule1/2(in_2), Rule2/2(in_2), Rule3/2(in_2), Rule4/2(in_2), Rule5/2(in_2), Rule7/2(in_2), Rule6/2(in_2)

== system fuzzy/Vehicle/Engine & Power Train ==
  theta : Inport  Port=1  PortWidth=-1  SampleTime=-1
  Acceleration constant : Gain  Gain=1/te_p
  Deceleration constant : Gain  Gain=1/te_n
  Discrete Derivative : Subsystem
  Engine Force : Fcn  Expr=Fi+gamma*sqrt(u[1])-gamma1*u[1]-gamma3*u[1]*u[1]*u[1]
  Integrator : Integrator  ExternalReset=none  InitialConditionSource=internal  InitialCondition=Fe0  LimitOutput=off  UpperSaturationLimit=inf  LowerSaturationLimit=-inf  ShowSaturationPort=off  ShowStatePort=off  AbsoluteTolerance=auto
  Sum : Sum  Inputs=-+
  Switch : Switch  Threshold=0
  Engine Force_ : Outport  Port=1  InitialOutput=0
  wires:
  theta/1 -> Discrete Derivative/1(e), Engine Force/1
  Discrete Derivative/1(ce) -> Switch/2
  Sum/1 -> Acceleration constant/1, Deceleration constant/1
  Acceleration constant/1 -> Switch/1
  Deceleration constant/1 -> Switch/3
  Switch/1 -> Integrator/1
  Integrator/1 -> Engine Force_/1, Sum/1
  Engine Force/1 -> Sum/2

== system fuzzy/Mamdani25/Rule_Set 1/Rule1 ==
  e_n : Inport  Port=1  PortWidth=-1  SampleTime=-1
  ce_n : Inport  Port=2  PortWidth=-1  SampleTime=-1
  LP(ce_n) : Lookup  InputValues=ce_n  OutputValues=LP
  LP(delta_u_n) : Constant  Value=uLP
  LP(e_n) : Lookup  InputValues=e_n  OutputValues=LP
  Product : Product  Inputs=2
  Product1 : Product  Inputs=2
  delta_u_n : Outport  Port=1  InitialOutput=0
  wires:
  Product1/1 -> delta_u_n/1
  LP(delta_u_n)/1 -> Product1/2
  Product/1 -> Product1/1
  ce_n/1 -> LP(ce_n)/1
  e_n/1 -> LP(e_n)/1
  LP(ce_n)/1 -> Product/2
  LP(e_n)/1 -> Product/1

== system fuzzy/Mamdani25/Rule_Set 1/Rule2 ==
  e_n : Inport  Port=1  PortWidth=-1  SampleTime=-1
  ce_n : Inport  Port=2  PortWidth=-1  SampleTime=-1
  Product : Product  Inputs=2
  Product1 : Product  Inputs=2
  SP(ce_n) : Lookup  InputValues=ce_n  OutputValues=SP
  SP(delta_u_n) : Constant  Value=uSP
  SP(e_n) : Lookup  InputValues=e_n  OutputValues=SP
  delta_u_n : Outport  Port=1  InitialOutput=0
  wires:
  SP(e_n)/1 -> Product/1
  SP(ce_n)/1 -> Product/2
  e_n/1 -> SP(e_n)/1
  ce_n/1 -> SP(ce_n)/1
  Product/1 -> Product1/1
  SP(delta_u_n)/1 -> Product1/2
  Product1/1 -> delta_u_n/1

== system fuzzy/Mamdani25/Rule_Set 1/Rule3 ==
  e_n : Inport  Port=1  PortWidth=-1  SampleTime=-1
  ce_n : Inport  Port=2  PortWidth=-1  SampleTime=-1
  Product : Product  Inputs=2
  Product1 : Product  Inputs=2
  SN(ce_n) : Lookup  InputValues=ce_n  OutputValues=SN
  SN(delta_u_n) : Constant  Value=uSN
  SN(e_n) : Lookup  InputValues=e_n  OutputValues=SN
  delta_u_n : Outport  Port=1  InitialOutput=0
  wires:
  Product1/1 -> delta_u_n/1
  SN(delta_u_n)/1 -> Product1/2
  Product/1 -> Product1/1
  ce_n/1 -> SN(ce_n)/1
  e_n/1 -> SN(e_n)/1
  SN(ce_n)/1 -> Product/2
  SN(e_n)/1 -> Product/1

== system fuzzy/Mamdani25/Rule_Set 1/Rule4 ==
  e_n : Inport  Port=1  PortWidth=-1  SampleTime=-1
  ce_n : Inport  Port=2  PortWidth=-1  SampleTime=-1
  LN(ce_n) : Lookup  InputValues=ce_n  OutputValues=LN
  LN(delta_u_n) : Constant  Value=uLN
  LN(e_n) : Lookup  InputValues=e_n  OutputValues=LN
  Product : Product  Inputs=2
  Product1 : Product  Inputs=2
  delta_u_n : Outport  Port=1  InitialOutput=0
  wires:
  LN(e_n)/1 -> Product/1
  LN(ce_n)/1 -> Product/2
  e_n/1 -> LN(e_n)/1
  ce_n/1 -> LN(ce_n)/1
  Product/1 -> Product1/1
  LN(delta_u_n)/1 -> Product1/2
  Product1/1 -> delta_u_n/1

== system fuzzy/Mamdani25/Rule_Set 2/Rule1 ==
  e_n : Inport  Port=1  PortWidth=-1  SampleTime=-1
  ce_n : Inport  Port=2  PortWidth=-1  SampleTime=-1
  LP(delta_u_n) : Constant  Value=uLP
  LP(e_n) : Lookup  InputValues=e_n  OutputValues=LP
  Product : Product  Inputs=2
  Product1 : Product  Inputs=2
  Z(ce_n) : Lookup  InputValues=ce_n  OutputValues=Z
  delta_u_n : Outport  Port=1  InitialOutput=0
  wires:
  LP(e_n)/1 -> Product/1
  Z(ce_n)/1 -> Product/2
  e_n/1 -> LP(e_n)/1
  ce_n/1 -> Z(ce_n)/1
  Product/1 -> Product1/1
  LP(delta_u_n)/1 -> Product1/2
  Product1/1 -> delta_u_n/1

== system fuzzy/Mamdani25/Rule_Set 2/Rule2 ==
  e_n : Inport  Port=1  PortWidth=-1  SampleTime=-1
  ce_n : Inport  Port=2  PortWidth=-1  SampleTime=-1
  Product : Product  Inputs=2
  Product1 : Product  Inputs=2
  SP(delta_u_n) : Constant  Value=uSP
  SP(e_n) : Lookup  InputValues=e_n  OutputValues=SP
  Z(ce_n) : Lookup  InputValues=ce_n  OutputValues=Z
  delta_u_n : Outport  Port=1  InitialOutput=0
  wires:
  Product1/1 -> delta_u_n/1
  SP(delta_u_n)/1 -> Product1/2
  Product/1 -> Product1/1
  ce_n/1 -> Z(ce_n)/1
  e_n/1 -> SP(e_n)/1
  Z(ce_n)/1 -> Product/2
  SP(e_n)/1 -> Product/1

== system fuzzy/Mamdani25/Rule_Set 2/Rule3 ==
  e_n : Inport  Port=1  PortWidth=-1  SampleTime=-1
  ce_n : Inport  Port=2  PortWidth=-1  SampleTime=-1
  Product : Product  Inputs=2
  Product1 : Product  Inputs=2
  SN(_ne) : Lookup  InputValues=e_n  OutputValues=SN
  SN(delta_u_n) : Constant  Value=uSN
  Z(ce_n) : Lookup  InputValues=ce_n  OutputValues=Z
  delta_u_n : Outport  Port=1  InitialOutput=0
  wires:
  SN(_ne)/1 -> Product/1
  Z(ce_n)/1 -> Product/2
  e_n/1 -> SN(_ne)/1
  ce_n/1 -> Z(ce_n)/1
  Product/1 -> Product1/1
  SN(delta_u_n)/1 -> Product1/2
  Product1/1 -> delta_u_n/1

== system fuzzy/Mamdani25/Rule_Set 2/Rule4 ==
  e_n : Inport  Port=1  PortWidth=-1  SampleTime=-1
  ce_n : Inport  Port=2  PortWidth=-1  SampleTime=-1
  LN(delta_u_n) : Constant  Value=uLN
  LN(e_n) : Lookup  InputValues=e_n  OutputValues=LN
  Product : Product  Inputs=2
  Product1 : Product  Inputs=2
  Z(ce_n) : Lookup  InputValues=ce_n  OutputValues=Z
  delta_u_n : Outport  Port=1  InitialOutput=0
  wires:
  Product1/1 -> delta_u_n/1
  LN(delta_u_n)/1 -> Product1/2
  Product/1 -> Product1/1
  ce_n/1 -> Z(ce_n)/1
  e_n/1 -> LN(e_n)/1
  Z(ce_n)/1 -> Product/2
  LN(e_n)/1 -> Product/1

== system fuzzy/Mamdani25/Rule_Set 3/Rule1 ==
  e_n : Inport  Port=1  PortWidth=-1  SampleTime=-1
  ce_n : Inport  Port=2  PortWidth=-1  SampleTime=-1
  LP(e_n) : Lookup  InputValues=e_n  OutputValues=LP
  Product : Product  Inputs=2
  Product1 : Product  Inputs=2
  SN(ce_n) : Lookup  InputValues=ce_n  OutputValues=SN
  Z(delta_u_n) : Constant  Value=uZ
  delta_u_n : Outport  Port=1  InitialOutput=0
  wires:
  Product1/1 -> delta_u_n/1
  Z(delta_u_n)/1 -> Product1/2
  Product/1 -> Product1/1
  ce_n/1 -> SN(ce_n)/1
  e_n/1 -> LP(e_n)/1
  SN(ce_n)/1 -> Product/2
  LP(e_n)/1 -> Product/1

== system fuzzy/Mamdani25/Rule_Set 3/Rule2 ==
  e_n : Inport  Port=1  PortWidth=-1  SampleTime=-1
  ce_n : Inport  Port=2  PortWidth=-1  SampleTime=-1
  Product : Product  Inputs=2
  Product1 : Product  Inputs=2
  SN(ce_n) : Lookup  InputValues=ce_n  OutputValues=SN
  SP(e_n) : Lookup  InputValues=e_n  OutputValues=SP
  Z(delta_u_n) : Constant  Value=uZ
  delta_u_n : Outport  Port=1  InitialOutput=0
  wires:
  SP(e_n)/1 -> Product/1
  SN(ce_n)/1 -> Product/2
  e_n/1 -> SP(e_n)/1
  ce_n/1 -> SN(ce_n)/1
  Product/1 -> Product1/1
  Z(delta_u_n)/1 -> Product1/2
  Product1/1 -> delta_u_n/1

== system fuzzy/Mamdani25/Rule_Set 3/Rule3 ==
  e_n : Inport  Port=1  PortWidth=-1  SampleTime=-1
  ce_n : Inport  Port=2  PortWidth=-1  SampleTime=-1
  Product : Product  Inputs=2
  Product1 : Product  Inputs=2
  SN(e_n) : Lookup  InputValues=e_n  OutputValues=SN
  SP(ce_n) : Lookup  InputValues=ce_n  OutputValues=SP
  Z(delta_u_n) : Constant  Value=uZ
  delta_u_n : Outport  Port=1  InitialOutput=0
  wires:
  Product1/1 -> delta_u_n/1
  Z(delta_u_n)/1 -> Product1/2
  Product/1 -> Product1/1
  ce_n/1 -> SP(ce_n)/1
  e_n/1 -> SN(e_n)/1
  SP(ce_n)/1 -> Product/2
  SN(e_n)/1 -> Product/1

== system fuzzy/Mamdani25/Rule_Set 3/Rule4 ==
  e_n : Inport  Port=1  PortWidth=-1  SampleTime=-1
  ce_n : Inport  Port=2  PortWidth=-1  SampleTime=-1
  LN(e_n) : Lookup  InputValues=e_n  OutputValues=LN
  Product : Product  Inputs=2
  Product1 : Product  Inputs=2
  SP(ce_n) : Lookup  InputValues=ce_n  OutputValues=SP
  Z(delta_u_n) : Constant  Value=uZ
  delta_u_n : Outport  Port=1  InitialOutput=0
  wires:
  LN(e_n)/1 -> Product/1
  SP(ce_n)/1 -> Product/2
  e_n/1 -> LN(e_n)/1
  ce_n/1 -> SP(ce_n)/1
  Product/1 -> Product1/1
  Z(delta_u_n)/1 -> Product1/2
  Product1/1 -> delta_u_n/1

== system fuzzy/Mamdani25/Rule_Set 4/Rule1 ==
  e_n : Inport  Port=1  PortWidth=-1  SampleTime=-1
  ce_n : Inport  Port=2  PortWidth=-1  SampleTime=-1
  LP(delta_u_n) : Constant  Value=uLP
  LP(e_n) : Lookup  InputValues=e_n  OutputValues=LP
  Product : Product  Inputs=2
  Product1 : Product  Inputs=2
  SP(ce_n) : Lookup  InputValues=ce_n  OutputValues=SP
  delta_u_n : Outport  Port=1  InitialOutput=0
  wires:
  LP(e_n)/1 -> Product/1
  SP(ce_n)/1 -> Product/2
  e_n/1 -> LP(e_n)/1
  ce_n/1 -> SP(ce_n)/1
  Product/1 -> Product1/1
  LP(delta_u_n)/1 -> Product1/2
  Product1/1 -> delta_u_n/1

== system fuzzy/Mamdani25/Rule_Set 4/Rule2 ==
  e_n : Inport  Port=1  PortWidth=-1  SampleTime=-1
  ce_n : Inport  Port=2  PortWidth=-1  SampleTime=-1
  LP(ce_n) : Lookup  InputValues=ce_n  OutputValues=LP
  LP(delta_u_n) : Constant  Value=uLP
  Product : Product  Inputs=2
  Product1 : Product  Inputs=2
  SP(e_n) : Lookup  InputValues=e_n  OutputValues=SP
  delta_u_n : Outport  Port=1  InitialOutput=0
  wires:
  Product1/1 -> delta_u_n/1
  LP(delta_u_n)/1 -> Product1/2
  Product/1 -> Product1/1
  ce_n/1 -> LP(ce_n)/1
  e_n/1 -> SP(e_n)/1
  LP(ce_n)/1 -> Product/2
  SP(e_n)/1 -> Product/1

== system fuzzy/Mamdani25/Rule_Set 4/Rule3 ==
  e_n : Inport  Port=1  PortWidth=-1  SampleTime=-1
  ce_n : Inport  Port=2  PortWidth=-1  SampleTime=-1
  LN(ce_n) : Lookup  InputValues=ce_n  OutputValues=LN
  LN(delta_u_n) : Constant  Value=uLN
  Product : Product  Inputs=2
  Product1 : Product  Inputs=2
  SN(e_n) : Lookup  InputValues=e_n  OutputValues=SN
  delta_u_n : Outport  Port=1  InitialOutput=0
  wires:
  SN(e_n)/1 -> Product/1
  LN(ce_n)/1 -> Product/2
  e_n/1 -> SN(e_n)/1
  ce_n/1 -> LN(ce_n)/1
  Product/1 -> Product1/1
  LN(delta_u_n)/1 -> Product1/2
  Product1/1 -> delta_u_n/1

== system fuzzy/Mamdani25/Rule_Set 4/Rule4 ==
  e_n : Inport  Port=1  PortWidth=-1  SampleTime=-1
  ce_n : Inport  Port=2  PortWidth=-1  SampleTime=-1
  LN(delta_u_n) : Constant  Value=uLN
  LN(e_n) : Lookup  InputValues=e_n  OutputValues=LN
  Product : Product  Inputs=2
  Product1 : Product  Inputs=2
  SN(ce_n) : Lookup  InputValues=ce_n  OutputValues=SN
  delta_u_n : Outport  Port=1  InitialOutput=0
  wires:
  Product1/1 -> delta_u_n/1
  LN(delta_u_n)/1 -> Product1/2
  Product/1 -> Product1/1
  ce_n/1 -> SN(ce_n)/1
  e_n/1 -> LN(e_n)/1
  SN(ce_n)/1 -> Product/2
  LN(e_n)/1 -> Product/1

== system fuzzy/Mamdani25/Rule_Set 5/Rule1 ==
  e_n : Inport  Port=1  PortWidth=-1  SampleTime=-1
  ce_n : Inport  Port=2  PortWidth=-1  SampleTime=-1
  LN(ce_n) : Lookup  InputValues=ce_n  OutputValues=LN
  LP(e_n) : Lookup  InputValues=e_n  OutputValues=LP
  Product : Product  Inputs=2
  Product1 : Product  Inputs=2
  SN(delta_u_n) : Constant  Value=uSN
  delta_u_n : Outport  Port=1  InitialOutput=0
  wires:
  Product1/1 -> delta_u_n/1
  SN(delta_u_n)/1 -> Product1/2
  Product/1 -> Product1/1
  ce_n/1 -> LN(ce_n)/1
  e_n/1 -> LP(e_n)/1
  LN(ce_n)/1 -> Product/2
  LP(e_n)/1 -> Product/1

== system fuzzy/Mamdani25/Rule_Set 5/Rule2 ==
  e_n : Inport  Port=1  PortWidth=-1  SampleTime=-1
  ce_n : Inport  Port=2  PortWidth=-1  SampleTime=-1
  LN(ce_n) : Lookup  InputValues=ce_n  OutputValues=LN
  Product : Product  Inputs=2
  Product1 : Product  Inputs=2
  SN(delta_u_n) : Constant  Value=uSN
  SP(e_n) : Lookup  InputValues=e_n  OutputValues=SP
  delta_u_n : Outport  Port=1  InitialOutput=0
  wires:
  SP(e_n)/1 -> Product/1
  LN(ce_n)/1 -> Product/2
  e_n/1 -> SP(e_n)/1
  ce_n/1 -> LN(ce_n)/1
  Product/1 -> Product1/1
  SN(delta_u_n)/1 -> Product1/2
  Product1/1 -> delta_u_n/1

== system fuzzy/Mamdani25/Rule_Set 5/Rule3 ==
  e_n : Inport  Port=1  PortWidth=-1  SampleTime=-1
  ce_n : Inport  Port=2  PortWidth=-1  SampleTime=-1
  LP(ce_n) : Lookup  InputValues=ce_n  OutputValues=LP
  Product : Product  Inputs=2
  Product1 : Product  Inputs=2
  SN(e_n) : Lookup  InputValues=e_n  OutputValues=SN
  SP(delta_u_n) : Constant  Value=uSP
  delta_u_n : Outport  Port=1  InitialOutput=0
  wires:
  Product1/1 -> delta_u_n/1
  SP(delta_u_n)/1 -> Product1/2
  Product/1 -> Product1/1
  ce_n/1 -> LP(ce_n)/1
  e_n/1 -> SN(e_n)/1
  LP(ce_n)/1 -> Product/2
  SN(e_n)/1 -> Product/1

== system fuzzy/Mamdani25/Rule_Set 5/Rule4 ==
  e_n : Inport  Port=1  PortWidth=-1  SampleTime=-1
  ce_n : Inport  Port=2  PortWidth=-1  SampleTime=-1
  LN(e_n) : Lookup  InputValues=e_n  OutputValues=LN
  LP(ce_n) : Lookup  InputValues=ce_n  OutputValues=LP
  Product : Product  Inputs=2
  Product1 : Product  Inputs=2
  SP(delta_u_n) : Constant  Value=uSP
  delta_u_n : Outport  Port=1  InitialOutput=0
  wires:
  LN(e_n)/1 -> Product/1
  LP(ce_n)/1 -> Product/2
  e_n/1 -> LN(e_n)/1
  ce_n/1 -> LP(ce_n)/1
  Product/1 -> Product1/1
  SP(delta_u_n)/1 -> Product1/2
  Product1/1 -> delta_u_n/1

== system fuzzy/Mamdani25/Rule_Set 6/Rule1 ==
  e_n : Inport  Port=1  PortWidth=-1  SampleTime=-1
  ce_n : Inport  Port=2  PortWidth=-1  SampleTime=-1
  Product : Product  Inputs=2
  Product1 : Product  Inputs=2
  Z(ce_n) : Lookup  InputValues=ce_n  OutputValues=Z
  Z(delta_u_n) : Constant  Value=uZ
  Z(e_n) : Lookup  InputValues=e_n  OutputValues=Z
  delta_u_n : Outport  Port=1  InitialOutput=0
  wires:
  Z(e_n)/1 -> Product/1
  Z(ce_n)/1 -> Product/2
  e_n/1 -> Z(e_n)/1
  ce_n/1 -> Z(ce_n)/1
  Product/1 -> Product1/1
  Z(delta_u_n)/1 -> Product1/2
  Product1/1 -> delta_u_n/1

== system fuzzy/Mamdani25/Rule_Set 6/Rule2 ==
  e_n : Inport  Port=1  PortWidth=-1  SampleTime=-1
  ce_n : Inport  Port=2  PortWidth=-1  SampleTime=-1
  Product : Product  Inputs=2
  Product1 : Product  Inputs=2
  SN(ce_n) : Lookup  InputValues=ce_n  OutputValues=SN
  Z(delta_u_n) : Constant  Value=uZ
  Z(e_n) : Lookup  InputValues=e_n  OutputValues=Z
  delta_u_n : Outport  Port=1  InitialOutput=0
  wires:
  Product1/1 -> delta_u_n/1
  Z(delta_u_n)/1 -> Product1/2
  Product/1 -> Product1/1
  ce_n/1 -> SN(ce_n)/1
  e_n/1 -> Z(e_n)/1
  SN(ce_n)/1 -> Product/2
  Z(e_n)/1 -> Product/1

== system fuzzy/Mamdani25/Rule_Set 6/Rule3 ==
  e_n : Inport  Port=1  PortWidth=-1  SampleTime=-1
  ce_n : Inport  Port=2  PortWidth=-1  SampleTime=-1
  Product : Product  Inputs=2
  Product1 : Product  Inputs=2
  SP(ce_n) : Lookup  InputValues=ce_n  OutputValues=SP
  Z(delta_u_n) : Constant  Value=uZ
  Z(e_n) : Lookup  InputValues=e_n  OutputValues=Z
  delta_u_n : Outport  Port=1  InitialOutput=0
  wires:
  Z(e_n)/1 -> Product/1
  SP(ce_n)/1 -> Product/2
  e_n/1 -> Z(e_n)/1
  ce_n/1 -> SP(ce_n)/1
  Product/1 -> Product1/1
  Z(delta_u_n)/1 -> Product1/2
  Product1/1 -> delta_u_n/1

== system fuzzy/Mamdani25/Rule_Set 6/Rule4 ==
  e_n : Inport  Port=1  PortWidth=-1  SampleTime=-1
  ce_n : Inport  Port=2  PortWidth=-1  SampleTime=-1
  Product : Product  Inputs=2
  Product1 : Product  Inputs=2
  SP(delta_u_n) : Constant  Value=uSP
  Z(e_n) : Lookup  InputValues=e_n  OutputValues=Z
  ZP(ce_n) : Lookup  InputValues=ce_n  OutputValues=LP
  delta_u_n : Outport  Port=1  InitialOutput=0
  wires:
  Product1/1 -> delta_u_n/1
  SP(delta_u_n)/1 -> Product1/2
  Product/1 -> Product1/1
  ce_n/1 -> ZP(ce_n)/1
  e_n/1 -> Z(e_n)/1
  ZP(ce_n)/1 -> Product/2
  Z(e_n)/1 -> Product/1

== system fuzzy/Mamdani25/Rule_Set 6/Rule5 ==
  e_n : Inport  Port=1  PortWidth=-1  SampleTime=-1
  ce_n : Inport  Port=2  PortWidth=-1  SampleTime=-1
  LN(ce_n) : Lookup  InputValues=ce_n  OutputValues=LN
  Product : Product  Inputs=2
  Product1 : Product  Inputs=2
  SN(delta_u_n) : Constant  Value=uSN
  Z(e_n) : Lookup  InputValues=e_n  OutputValues=Z
  delta_u_n : Outport  Port=1  InitialOutput=0
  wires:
  Z(e_n)/1 -> Product/1
  LN(ce_n)/1 -> Product/2
  e_n/1 -> Z(e_n)/1
  ce_n/1 -> LN(ce_n)/1
  Product/1 -> Product1/1
  SN(delta_u_n)/1 -> Product1/2
  Product1/1 -> delta_u_n/1

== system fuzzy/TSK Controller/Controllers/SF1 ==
  e_n : Inport  Port=1  PortWidth=-1  SampleTime=-1
  ce_n : Inport  Port=2  PortWidth=-1  SampleTime=-1
  K10 : Constant  Value=K0
  K11 : Gain  Gain=K1
  K12 : Gain  Gain=K2
  Sum : Sum  Inputs=+++
  delta_u_n1 : Outport  Port=1  InitialOutput=0
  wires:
  K10/1 -> Sum/3
  K11/1 -> Sum/1
  K12/1 -> Sum/2
  e_n/1 -> K11/1
  Sum/1 -> delta_u_n1/1
  ce_n/1 -> K12/1

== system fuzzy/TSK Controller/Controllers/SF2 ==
  in_1 : Inport  Port=1  PortWidth=-1  SampleTime=-1
  in_2 : Inport  Port=2  PortWidth=-1  SampleTime=-1
  Constant : Constant  Value=K0
  K1 : Gain  Gain=K1
  K2 : Gain  Gain=K2
  Sum : Sum  Inputs=+++
  out_1 : Outport  Port=1  InitialOutput=0
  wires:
  in_2/1 -> K2/1
  Sum/1 -> out_1/1
  in_1/1 -> K1/1
  K2/1 -> Sum/2
  K1/1 -> Sum/1
  Constant/1 -> Sum/3

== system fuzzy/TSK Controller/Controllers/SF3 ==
  in_1 : Inport  Port=1  PortWidth=-1  SampleTime=-1
  in_2 : Inport  Port=2  PortWidth=-1  SampleTime=-1
  Constant : Constant  Value=K0
  K1 : Gain  Gain=K1
  K2 : Gain  Gain=K2
  Sum : Sum  Inputs=+++
  out_1 : Outport  Port=1  InitialOutput=0
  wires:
  Constant/1 -> Sum/3
  K1/1 -> Sum/1
  K2/1 -> Sum/2
  in_1/1 -> K1/1
  Sum/1 -> out_1/1
  in_2/1 -> K2/1

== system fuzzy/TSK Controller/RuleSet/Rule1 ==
  in_1 : Inport  Port=1  PortWidth=-1  SampleTime=-1
  in_2 : Inport  Port=2  PortWidth=-1  SampleTime=-1
  Product1 : Product  Inputs=2
  S : Lookup  InputValues=e_n  OutputValues=N
  any : Lookup  InputValues=ce_n  OutputValues=any
  out_1 : Outport  Port=1  InitialOutput=0
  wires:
  any/1 -> Product1/2
  S/1 -> Product1/1
  in_1/1 -> S/1
  Product1/1 -> out_1/1
  in_2/1 -> any/1

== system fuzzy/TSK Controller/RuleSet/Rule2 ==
  in_1 : Inport  Port=1  PortWidth=-1  SampleTime=-1
  in_2 : Inport  Port=2  PortWidth=-1  SampleTime=-1
  Product1 : Product  Inputs=2
  Z : Lookup  InputValues=e_n  OutputValues=Z
  any : Lookup  InputValues=ce_n  OutputValues=any
  out_1 : Outport  Port=1  InitialOutput=0
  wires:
  in_2/1 -> any/1
  Product1/1 -> out_1/1
  in_1/1 -> Z/1
  Z/1 -> Product1/1
  any/1 -> Product1/2

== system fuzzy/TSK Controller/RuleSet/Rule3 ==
  in_1 : Inport  Port=1  PortWidth=-1  SampleTime=-1
  in_2 : Inport  Port=2  PortWidth=-1  SampleTime=-1
  P : Lookup  InputValues=e_n  OutputValues=P
  Product1 : Product  Inputs=2
  any : Lookup  InputValues=ce_n  OutputValues=any
  out_1 : Outport  Port=1  InitialOutput=0
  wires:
  any/1 -> Product1/2
  P/1 -> Product1/1
  in_1/1 -> P/1
  Product1/1 -> out_1/1
  in_2/1 -> any/1

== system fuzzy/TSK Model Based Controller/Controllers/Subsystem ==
  in_1 : Inport  Port=1  PortWidth=-1  SampleTime=-1
  in_2 : Inport  Port=2  PortWidth=-1  SampleTime=-1
  Constant : Constant  Value=K0
  K1 : Gain  Gain=K1
  K2 : Gain  Gain=K2
  Sum : Sum  Inputs=+++
  out_1 : Outport  Port=1  InitialOutput=0
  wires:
  in_2/1 -> K2/1
  Sum/1 -> out_1/1
  in_1/1 -> K1/1
  K2/1 -> Sum/2
  K1/1 -> Sum/1
  Constant/1 -> Sum/3

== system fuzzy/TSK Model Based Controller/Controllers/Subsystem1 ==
  in_1 : Inport  Port=1  PortWidth=-1  SampleTime=-1
  in_2 : Inport  Port=2  PortWidth=-1  SampleTime=-1
  Constant : Constant  Value=K0
  K1 : Gain  Gain=K1
  K2 : Gain  Gain=K2
  Sum : Sum  Inputs=+++
  out_1 : Outport  Port=1  InitialOutput=0
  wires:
  Constant/1 -> Sum/3
  K1/1 -> Sum/1
  K2/1 -> Sum/2
  in_1/1 -> K1/1
  Sum/1 -> out_1/1
  in_2/1 -> K2/1

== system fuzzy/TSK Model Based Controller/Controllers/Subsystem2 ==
  in_1 : Inport  Port=1  PortWidth=-1  SampleTime=-1
  in_2 : Inport  Port=2  PortWidth=-1  SampleTime=-1
  Constant : Constant  Value=K0
  K1 : Gain  Gain=K1
  K2 : Gain  Gain=K2
  Sum : Sum  Inputs=+++
  out_1 : Outport  Port=1  InitialOutput=0
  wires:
  in_2/1 -> K2/1
  Sum/1 -> out_1/1
  in_1/1 -> K1/1
  K2/1 -> Sum/2
  K1/1 -> Sum/1
  Constant/1 -> Sum/3

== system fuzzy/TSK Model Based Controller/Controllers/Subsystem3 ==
  in_1 : Inport  Port=1  PortWidth=-1  SampleTime=-1
  in_2 : Inport  Port=2  PortWidth=-1  SampleTime=-1
  Constant : Constant  Value=K0
  K1 : Gain  Gain=K1
  K2 : Gain  Gain=K2
  Sum : Sum  Inputs=+++
  out_1 : Outport  Port=1  InitialOutput=0
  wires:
  Constant/1 -> Sum/3
  K1/1 -> Sum/1
  K2/1 -> Sum/2
  in_1/1 -> K1/1
  Sum/1 -> out_1/1
  in_2/1 -> K2/1

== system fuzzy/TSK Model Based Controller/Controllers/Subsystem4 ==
  in_1 : Inport  Port=1  PortWidth=-1  SampleTime=-1
  in_2 : Inport  Port=2  PortWidth=-1  SampleTime=-1
  Constant : Constant  Value=K0
  K1 : Gain  Gain=K1
  K2 : Gain  Gain=K2
  Sum : Sum  Inputs=+++
  out_1 : Outport  Port=1  InitialOutput=0
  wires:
  in_2/1 -> K2/1
  Sum/1 -> out_1/1
  in_1/1 -> K1/1
  K2/1 -> Sum/2
  K1/1 -> Sum/1
  Constant/1 -> Sum/3

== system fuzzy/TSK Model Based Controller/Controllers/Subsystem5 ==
  in_1 : Inport  Port=1  PortWidth=-1  SampleTime=-1
  in_2 : Inport  Port=2  PortWidth=-1  SampleTime=-1
  Constant : Constant  Value=K0
  K1 : Gain  Gain=K1
  K2 : Gain  Gain=K2
  Sum : Sum  Inputs=+++
  out_1 : Outport  Port=1  InitialOutput=0
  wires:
  Constant/1 -> Sum/3
  K1/1 -> Sum/1
  K2/1 -> Sum/2
  in_1/1 -> K1/1
  Sum/1 -> out_1/1
  in_2/1 -> K2/1

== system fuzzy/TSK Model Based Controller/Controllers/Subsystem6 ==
  in_1 : Inport  Port=1  PortWidth=-1  SampleTime=-1
  in_2 : Inport  Port=2  PortWidth=-1  SampleTime=-1
  Constant : Constant  Value=K0
  K1 : Gain  Gain=K1
  K2 : Gain  Gain=K2
  Sum : Sum  Inputs=+++
  out_1 : Outport  Port=1  InitialOutput=0
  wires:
  in_2/1 -> K2/1
  Sum/1 -> out_1/1
  in_1/1 -> K1/1
  K2/1 -> Sum/2
  K1/1 -> Sum/1
  Constant/1 -> Sum/3

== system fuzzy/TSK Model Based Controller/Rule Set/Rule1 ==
  in_1 : Inport  Port=1  PortWidth=-1  SampleTime=-1
  in_2 : Inport  Port=2  PortWidth=-1  SampleTime=-1
  Product1 : Product  Inputs=2
  Zero : Lookup  InputValues=x  OutputValues=ze
  any : Lookup  InputValues=i1  OutputValues=any
  out_1 : Outport  Port=1  InitialOutput=0
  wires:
  any/1 -> Product1/2
  Zero/1 -> Product1/1
  in_1/1 -> Zero/1
  Product1/1 -> out_1/1
  in_2/1 -> any/1

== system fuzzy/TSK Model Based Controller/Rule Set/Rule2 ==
  in_1 : Inport  Port=1  PortWidth=-1  SampleTime=-1
  in_2 : Inport  Port=2  PortWidth=-1  SampleTime=-1
  PM : Lookup  InputValues=x  OutputValues=pm
  Product1 : Product  Inputs=2
  Z1 : Lookup  InputValues=i1  OutputValues=zi
  out_1 : Outport  Port=1  InitialOutput=0
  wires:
  in_2/1 -> Z1/1
  Product1/1 -> out_1/1
  in_1/1 -> PM/1
  PM/1 -> Product1/1
  Z1/1 -> Product1/2
